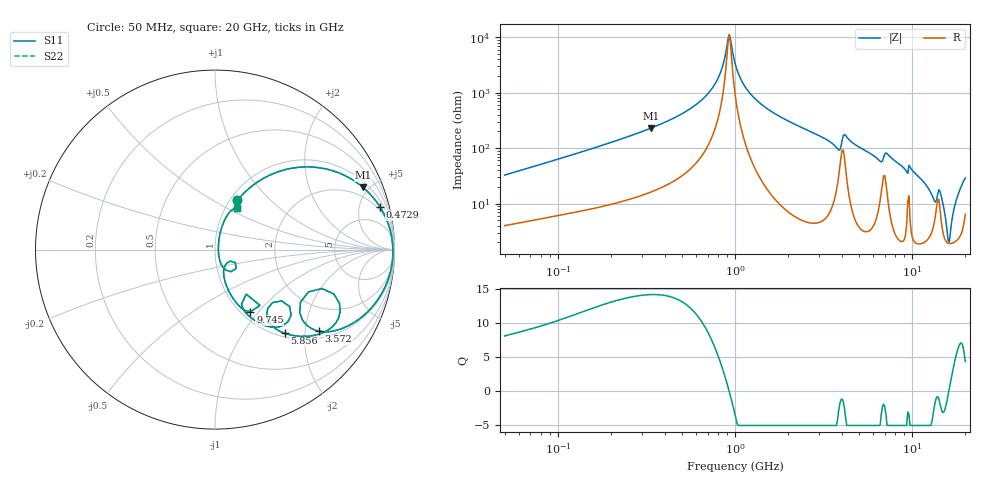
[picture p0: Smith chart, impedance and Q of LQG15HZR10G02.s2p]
!Murata Part Number: LQG15HZR10G02
!These Parameters are Measured in Series Mode Connection
!  o--[Z]--o
!Port1  Port2
!  o-------o
!Freq. Start=50[MHz] Stop=20[GHz], 401[Steps]
# Hz S RI R 50
!Freq.(Hz) S11(Real) S11(Imag) S21(Real) S21(Imag) S12(Real) S12(Imag) S22(Real) S22(Imag)
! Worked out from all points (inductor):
!   401 points, 50 MHz to 20 GHz, reference 50 ohm
!   read as one part in series: L = 102 nH near 51.52 MHz
!   highest Q = 14.2 at 335.1 MHz (marker M1), where L = 109 nH
!   self-resonance near 914 MHz
!   S11 on the Smith chart (normalised r, x): 50 MHz: 1.08, +0.65; 472.9 MHz: 1.56, +7.52; 3.572 GHz: 1.19, -2.37; 5.856 GHz: 1.07, -1.58; 9.745 GHz: 1.10, -0.91; 20 GHz: 1.13, +0.56
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5e7  0.1239 0.2736  0.8761 -0.2736  0.8761 -0.2736  0.1239 0.2736
1.364002e8  0.4307 0.454  0.5693 -0.454  0.5693 -0.454  0.4307 0.454
3.350611e8  0.8241 0.3471  0.1759 -0.3471  0.1759 -0.3471  0.8241 0.3471
3.721004e8  0.8575 0.316  0.1425 -0.316  0.1425 -0.316  0.8575 0.316
4.728708e8  0.9189 0.2384  0.0811 -0.2384  0.0811 -0.2384  0.9189 0.2384
7.411344e8  0.9822 0.081  0.0178 -0.081  0.0178 -0.081  0.9822 0.081
8.354841e8  0.9888 0.0378  0.0112 -0.0378  0.0112 -0.0378  0.9888 0.0378
9.278425e8  0.9912 -0.000206  0.00881 0.000206  0.00881 0.000206  0.9912 -0.000206
1e9  0.991 -0.0276  0.00902 0.0276  0.00902 0.0276  0.991 -0.0276
1.127304e9  0.9872 -0.0718  0.0128 0.0718  0.0128 0.0718  0.9872 -0.0718
1.349283e9  0.9732 -0.1391  0.0268 0.1391  0.0268 0.1391  0.9732 -0.1391
2.728004e9  0.7824 -0.4012  0.2176 0.4012  0.2176 0.4012  0.7824 -0.4012
3.572216e9  0.5801 -0.4547  0.4199 0.4547  0.4199 0.4547  0.5801 -0.4547
4.026975e9  0.5964 -0.2169  0.4036 0.2169  0.4036 0.2169  0.5964 -0.2169
5.856089e9  0.3882 -0.4661  0.6118 0.4661  0.6118 0.4661  0.3882 -0.4661
7.442007e9  0.3565 -0.4303  0.6435 0.4303  0.6435 0.4303  0.3565 -0.4303
9.745021e9  0.1975 -0.3465  0.8025 0.3465  0.8025 0.3465  0.1975 -0.3465
1.334722e10  0.0533 -0.0943  0.9467 0.0943  0.9467 0.0943  0.0533 -0.0943
1.438523e10  0.0896 -0.1229  0.9104 0.1229  0.9104 0.1229  0.0896 -0.1229
1.621653e10  0.0187 0.00663  0.9813 -0.00663  0.9813 -0.00663  0.0187 0.00663
1.800918e10  0.0376 0.1236  0.9624 -0.1236  0.9624 -0.1236  0.0376 0.1236
2e10  0.1219 0.2322  0.8781 -0.2322  0.8781 -0.2322  0.1219 0.2322
